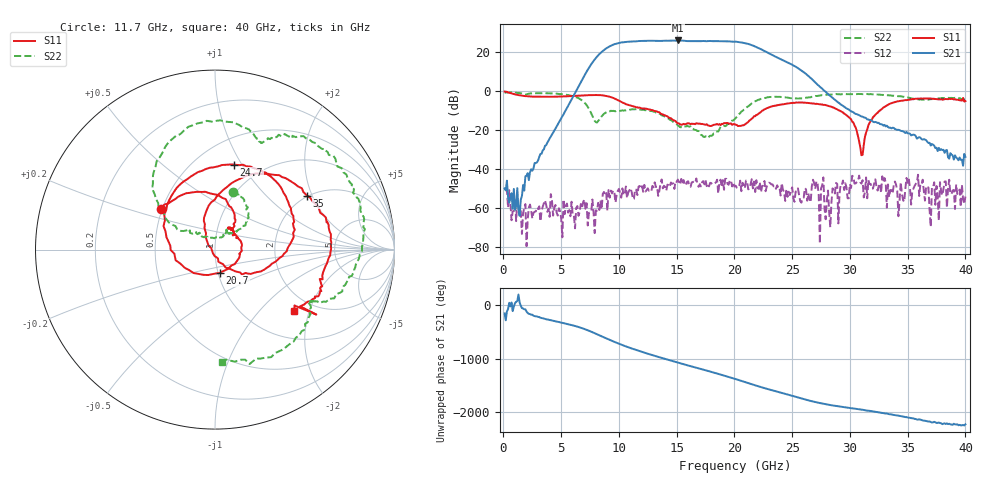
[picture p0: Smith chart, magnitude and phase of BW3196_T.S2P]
!Keysight Technologies,N5245A,MY52451660,A.10.49.11
!Date: Wednesday, January 24, 2018 10:25:16
!Correction: S11(Full 2 Port(1,2))
!S21(Full 2 Port(1,2))
!S12(Full 2 Port(1,2))
!S22(Full 2 Port(1,2))
!S2P File: Measurements: S11, S21, S12, S22:
# Hz S  dB  R 50
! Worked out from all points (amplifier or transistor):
!   400 points, 100 MHz to 40 GHz, reference 50 ohm
!   highest |S21| = 26.1 dB at 15.1 GHz (marker M1)
!   |S21| within 3 dB of that: 9.205 GHz to 21.74 GHz (12.54 GHz wide, 81 % of centre)
!   unconditionally stable (mu >= 1): start of sweep to end of sweep
!   at 6.7 GHz: K = 58.82, MAG = 10.6 dB, |S12| = -57.9 dB
!   at 20.1 GHz: K = 6.78, MAG = 25.7 dB, |S12| = -48.5 dB
!   at 40 GHz: K = 5220.89, MAG = -30.0 dB, |S12| = -54.2 dB
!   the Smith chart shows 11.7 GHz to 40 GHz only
!   S11 on the Smith chart (normalised r, x): 11.7 GHz: 0.49, +0.26; 20.7 GHz: 1.02, -0.27; 24.7 GHz: 0.75, +0.93; 35 GHz: 1.97, +1.83; 40 GHz: 1.61, -1.60
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1e8  -0.20 -12.6  -49.94 -157.6  -50.30 89.6  -0.70 178.6
6.8e9  -2.24 19.6  5.77 -70.8  -59.86 -100.1  -4.76 58.8
8.4e9  -2.03 -53.8  19.59 146.6  -56.57 -165.8  -13.71 97.7
9.2e9  -2.86 -100.2  23.05 70.3  -54.68 67.6  -10.41 94.6
1.01e10  -5.15 -150.9  24.90 -10.1  -52.29 40.9  -10.12 88.7
1.09e10  -7.21 173.5  25.45 -73.9  -51.00 -61.4  -9.56 83.0
1.17e10  -8.48 142.9  25.76 -131.8  -49.02 -99.6  -9.41 72.8
1.25e10  -9.22 113.7  25.88 172.6  -49.93 -157.8  -9.74 61.3
1.34e10  -10.71 82.1  25.86 114.0  -53.80 179.9  -11.07 47.8
1.51e10  -16.57 53.5  26.06 8.6  -45.40 86.1  -17.68 44.7
1.66e10  -16.95 51.3  25.72 -81.8  -47.06 22.4  -19.90 62.0
1.81e10  -17.59 39.5  25.72 -171.8  -47.88 -19.6  -22.68 117.1
1.92e10  -16.44 18.7  25.63 120.0  -45.05 -66.9  -17.99 135.3
2.01e10  -17.21 -27.9  25.46 62.3  -48.55 -102.4  -13.85 149.4
2.07e10  -17.50 -77.6  24.93 20.5  -47.03 -124.3  -10.11 148.4
2.21e10  -11.48 169.0  22.11 -75.0  -50.18 144.6  -4.41 120.5
2.33e10  -7.71 118.2  18.54 -149.5  -47.89 128.9  -2.87 93.7
2.47e10  -6.28 77.4  14.48 128.8  -51.64 79.1  -3.39 71.4
2.67e10  -6.26 32.8  6.26 9.0  -48.94 45.5  -2.88 61.2
3.34e10  -6.63 64.1  -18.76 128.0  -54.44 -69.1  -2.11 -8.5
3.5e10  -4.52 30.4  -21.68 67.6  -47.06 -27.0  -3.20 -23.9
4e10  -5.06 -37.6  -33.76 -61.6  -54.16 87.5  -4.08 -86.7
